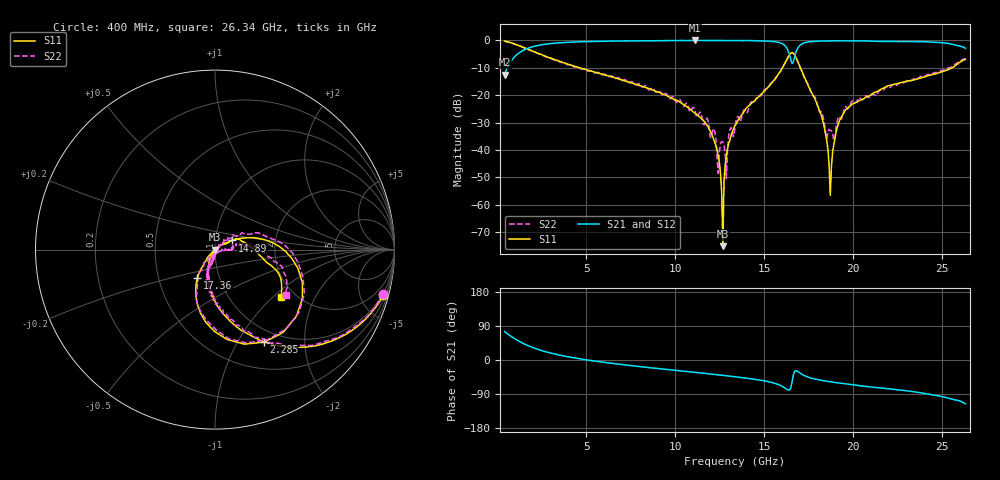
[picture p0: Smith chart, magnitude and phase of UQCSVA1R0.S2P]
!  Part Number  UQCSVA1R0  Mounting Orientation: Horizontal
!  Description: Ultra Low ESR Microwave capacitors
!  Application: Coupling, Bypass, Tuning, DC Block
!  Filters, Matching
# GHZ S DB R 50
! Freq  |S11|  S11 Ph  |S21|  S21 Ph  |S12|  S12 Ph  |S22|  S22 Ph
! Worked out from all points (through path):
!   400 points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, 400 MHz to 26.34 GHz, reference 50 ohm
!   highest |S21| = 0.00 dB at 11.12 GHz (marker M1); lowest = -12.6 dB at 400 MHz (marker M2)
!   group delay of S21, straight-line fit = 14.4 ps
!   lowest |S11| = -75.1 dB at 12.69 GHz (marker M3), VSWR 1.00, Z = 50 + j0.0127 ohm
!   |S11| at or under -10 dB: 4.641 GHz to 16.03 GHz (11.39 GHz wide, 110 % of centre); 17.05 GHz to 25.59 GHz (8.539 GHz wide, 40.1 % of centre)
!   |S22| runs from -50.4 to -0.3 dB; largest |S21 - S12| = 0.011
!   S11 on the Smith chart (normalised r, x): 400 MHz: 0.83, -7.50; 2.285 GHz: 0.84, -1.29; 14.89 GHz: 1.20, +0.13; 17.36 GHz: 0.79, -0.25; 26.34 GHz: 1.70, -1.13
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0.4  -0.25 -15.0  -12.55 74.7  -12.52 74.3  -0.28 -14.8
2.285  -4.73 -62.1  -1.82 27.9  -1.84 27.6  -4.79 -61.0
4.755  -10.24 -88.2  -0.46 2.1  -0.45 2.3  -10.47 -88.8
9.045  -18.83 -109.7  -0.08 -22.5  -0.07 -22.4  -18.36 -111.2
11.125  -26.64 -118.8  0.00 -32.6  -0.01 -32.7  -25.89 -93.8
12.36  -39.95 -125.7  -0.01 -38.8  -0.01 -39.0  -43.14 -42.4
12.62  -55.66 -132.4  -0.01 -40.2  -0.01 -40.3  -36.92 -42.0
12.685  -75.13 133.7  -0.01 -40.5  -0.01 -40.7  -37.11 -4.0
12.815  -45.46 56.3  0.00 -41.2  -0.01 -41.4  -40.93 63.8
12.88  -42.43 53.6  0.00 -41.5  -0.01 -41.7  -50.43 50.3
13.01  -37.61 52.7  -0.01 -42.3  0.00 -42.4  -35.03 11.8
13.4  -30.81 44.1  -0.02 -44.5  -0.03 -44.6  -30.10 31.6
14.895  -19.28 28.2  -0.16 -54.0  -0.14 -54.3  -19.53 36.1
16.585  -4.48 -50.7  -8.43 -56.8  -8.43 -56.9  -4.53 -48.2
17.365  -14.70 -122.0  -0.69 -43.1  -0.67 -43.5  -14.86 -122.7
17.69  -19.13 -126.8  -0.40 -48.2  -0.37 -48.6  -19.56 -126.3
18.47  -34.32 -136.3  -0.18 -55.6  -0.18 -56.0  -33.68 -97.9
18.73  -56.63 -48.8  -0.15 -57.5  -0.15 -58.0  -32.93 -62.0
18.86  -40.93 37.4  -0.14 -58.4  -0.15 -58.9  -33.77 -15.7
19.25  -29.25 39.4  -0.12 -60.8  -0.12 -61.4  -27.82 6.8
22.045  -16.47 20.8  -0.36 -76.0  -0.37 -76.6  -17.22 13.9
26.335  -6.87 -35.4  -2.87 -115.5  -2.87 -116.1  -6.57 -32.9
